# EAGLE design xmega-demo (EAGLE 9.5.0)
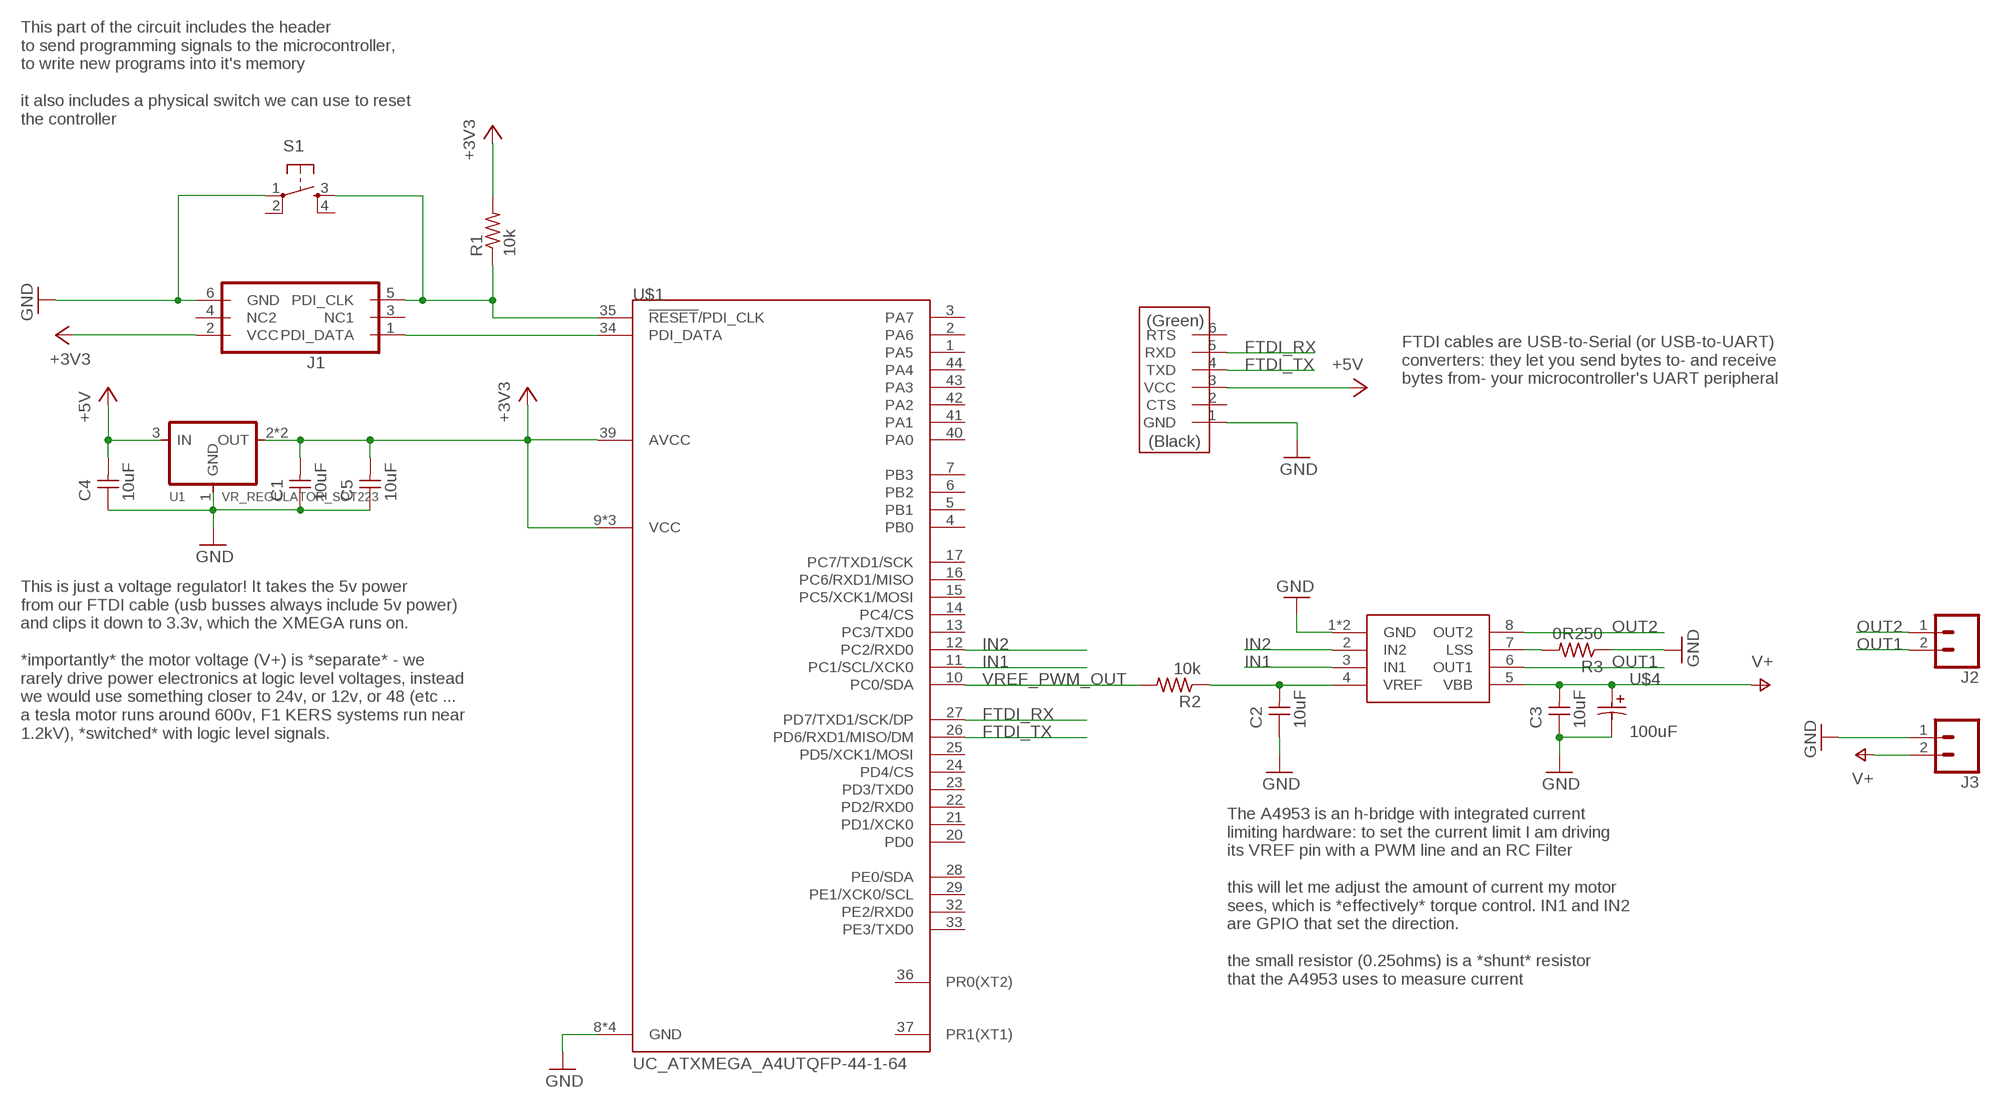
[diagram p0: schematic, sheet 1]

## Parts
C1  10uF  CAP_UNPOLARIZEDFAB  [C1206FAB]
C2  10uF  CAP_UNPOLARIZEDFAB  [C1206FAB]
C3  10uF  CAP_UNPOLARIZEDFAB  [C1206FAB]
C4  10uF  CAP_UNPOLARIZEDFAB  [C1206FAB]
C5  10uF  CAP_UNPOLARIZEDFAB  [C1206FAB]
J1  CONN_03X2_PDIFEMALE_SMD  [PDI_2X3_SMD]
J2  CONN_02  [1X02]
J3  CONN_02  [1X02]
R1  10k  R1206FAB  [R1206FAB]
R2  10k  R1206FAB  [R1206FAB]
R3  0R250  R1206FAB  [R1206FAB]
S1  SW_SWITCH_TACTILE_6MM6MM_SWITCH  [6MM_SWITCH]
U1  VR_REGULATOR_SOT223  [SOT223]
U$1  UC_ATXMEGA_A4UTQFP-44-1-64  [TQFP44-13THIN]
U$2  CONN_06_FTDI-SMD-HEADER  [1X06SMD]
U$3  PMIC_H-BRIDGE_A4953_PAD  [SOIC8_PAD]
U$4  100uF  CAP_POLARIZED  [SMD-ELEC-CAP]

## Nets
+3V3: C1.2 C5.2 J1.2(VCC) R1.2 U1.2(OUT) U1.4(OUT) U$1.9(VCC) U$1.19(VCC) U$1.31(VCC) U$1.39(AVCC)
+5V: C4.2 U1.3(IN) U$2.3(VCC)
FTDI_RX: U$1.27(PD7/TXD1/SCK/DP) U$2.5(RXD)
FTDI_TX: U$1.26(PD6/RXD1/MISO/DM) U$2.4(TXD)
GND: C1.1 C2.1 C3.1 C4.1 C5.1 J1.6(GND) J3.1 R3.1 S1.1(P) U1.1(GND) U$1.8(GND) U$1.18(GND) U$1.30(GND) U$1.38(GND) U$2.1(GND) U$3.1(GND) U$3.GND U$4.C
IN1: U$1.11(PC1/SCL/XCK0) U$3.3(IN1)
IN2: U$1.12(PC2/RXD0) U$3.2(IN2)
N$1: J1.1(PDI_DATA) U$1.34(PDI_DATA)
N$2: J1.5(PDI_CLK) R1.1 S1.3(S) U$1.35(!RESET!/PDI_CLK)
N$3: C2.2 R2.1 U$3.4(VREF)
N$5: R3.2 U$3.7(LSS)
OUT1: J2.2 U$3.6(OUT1)
OUT2: J2.1 U$3.8(OUT2)
V+: C3.2 J3.2 U$3.5(VBB) U$4.A
VREF_PWM_OUT: R2.2 U$1.10(PC0/SDA)
Unconnected: J1.3(NC1) J1.4(NC2) S1.2(P1) S1.4(S1) U$1.1(PA5) U$1.2(PA6) U$1.3(PA7) U$1.4(PB0) U$1.5(PB1) U$1.6(PB2) U$1.7(PB3) U$1.13(PC3/TXD0) U$1.14(PC4/CS) U$1.15(PC5/XCK1/MOSI) U$1.16(PC6/RXD1/MISO) U$1.17(PC7/TXD1/SCK) U$1.20(PD0) U$1.21(PD1/XCK0) U$1.22(PD2/RXD0) U$1.23(PD3/TXD0) U$1.24(PD4/CS) U$1.25(PD5/XCK1/MOSI) U$1.28(PE0/SDA) U$1.29(PE1/XCK0/SCL) U$1.32(PE2/RXD0) U$1.33(PE3/TXD0) U$1.36(PR0(XT2)) U$1.37(PR1(XT1)) U$1.40(PA0) U$1.41(PA1) U$1.42(PA2) U$1.43(PA3) U$1.44(PA4) U$2.2(CTS) U$2.6(RTS)

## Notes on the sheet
- This part of the circuit includes the header
  to send programming signals to the microcontroller,
  to write new programs into it's memory
  
  it also includes a physical switch we can use to reset 
  the controller
- FTDI cables are USB-to-Serial (or USB-to-UART) 
  converters: they let you send bytes to- and receive 
  bytes from- your microcontroller's UART peripheral
- This is just a voltage regulator! It takes the 5v power 
  from our FTDI cable (usb busses always include 5v power)
  and clips it down to 3.3v, which the XMEGA runs on.
  
  *importantly* the motor voltage (V+) is *separate* - we
  rarely drive power electronics at logic level voltages, instead
  we would use something closer to 24v, or 12v, or 48 (etc ...
  a tesla motor runs around 600v, F1 KERS systems run near 
  1.2kV), *switched* with logic level signals.
- The A4953 is an h-bridge with integrated current
  limiting hardware: to set the current limit I am driving 
  its VREF pin with a PWM line and an RC Filter
  
  this will let me adjust the amount of current my motor 
  sees, which is *effectively* torque control. IN1 and IN2 
  are GPIO that set the direction. 
  
  the small resistor (0.25ohms) is a *shunt* resistor
  that the A4953 uses to measure current

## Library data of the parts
C1-C5 = fablab:CAP_UNPOLARIZED
J1 = fablab:CONN_03X2_PDI: Multi connection point. Often used as Generic Header-pin footprint for 0.1 inch spaced/style header connections You can populate with any combo of single row headers, but if you'd like an exact match, check these: Header - 2x3 (Male, 0.1") (PRT-12807) Header - 2x3 (Female, 0.1") (PRT-13010) 2x3 Pin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; PROD_ID: CONN-11290
J2 J3 = SparkFun-Connectors:CONN_02: Multi connection point. Often used as Generic Header-pin footprint for 0.1 inch spaced/style header connections
R1-R3 = fablab:R: Resistor (US Symbol)
S1 = fablab:SW_SWITCH_TACTILE_6MM: OMRON SWITCH
U1 = fablab:VR_REGULATOR_SOT223
U$1 = fablab:UC_ATXMEGA_A4U
U$2 = fablab:CONN_06_FTDI-SMD-HEADER
U$3 = fablab:PMIC_H-BRIDGE_A4953_PAD
U$4 = fablab:CAP_POLARIZED

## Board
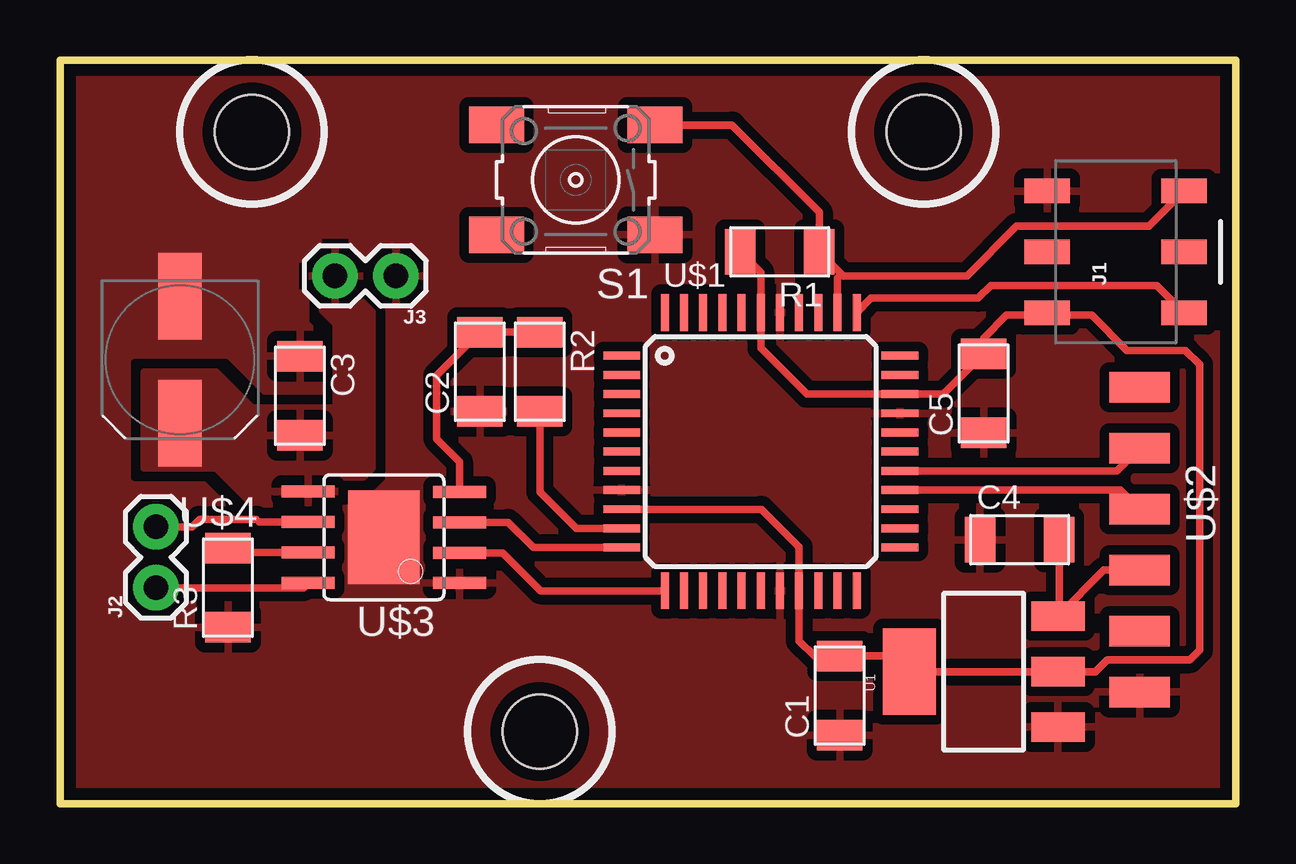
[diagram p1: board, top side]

Size 49 x 31 mm. Coordinates in mm from the lower left corner, seen from the top.
Outline: 0,0 49,0 49,31 0,31 0,0
Copper layers (1*16): Top 0.035mm / dielectric 1.5mm / Bottom 0.035mm
Design rules "default *": minimum track width 12mil, minimum drill 32mil, track to track 16mil, track to pad 16mil, pad to pad 16mil, via to via 16mil, smd to smd 0mil, copper to edge 20mil, drill to drill 16mil, minimum pad ring 10mil, minimum via ring 8mil, stop-mask expansion 4mil, vias tented up to drill 0mil, thermal gap 17mil
Holes 3.1 mm at 20,3 8,28 36,28

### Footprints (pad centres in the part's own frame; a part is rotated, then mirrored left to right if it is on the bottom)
C1206FAB = smd 1.27 x 1.905: 1 -1.651,0; 2 1.651,0
PDI_2X3_SMD = smd 1.02 x 1.9: 1 -2.54,-2.85; 2 -2.54,2.85; 3 0,-2.85; 4 0,2.85; 5 2.54,-2.85; 6 2.54,2.85
1X02 = drill 1.016 pad 1.88: 1 0,0; 2 2.54,0
R1206FAB = smd 1.27 x 1.905: 1 -1.651,0; 2 1.651,0
6MM_SWITCH = smd 2.286 x 1.524: 1 -3.302,2.286; 2 3.302,2.286; 3 -3.302,-2.286; 4 3.302,-2.286
SOT223 = smd 1.219 x 2.235: 1 -2.311,-3.099; 2 0,-3.099; 3 2.311,-3.099 | smd 3.6 x 2.2: 4 0,3.099
TQFP44-13THIN = smd 1.524 x 0.33: 1 -5.8,4; 2 -5.8,3.2; 3 -5.8,2.4; 4 -5.8,1.6; 5 -5.8,0.8; 6 -5.8,0; 7 -5.8,-0.8; 8 -5.8,-1.6; 9 -5.8,-2.4; 10 -5.8,-3.2; 11 -5.8,-4; 23 5.8,-4; 24 5.8,-3.2; 25 5.8,-2.4; 26 5.8,-1.6; 27 5.8,-0.8; 28 5.8,0; 29 5.8,0.8; 30 5.8,1.6; 31 5.8,2.4; 32 5.8,3.2; 33 5.8,4 | smd 0.33 x 1.524: 12 -4,-5.8; 13 -3.2,-5.8; 14 -2.4,-5.8; 15 -1.6,-5.8; 16 -0.8,-5.8; 17 0,-5.8; 18 0.8,-5.8; 19 1.6,-5.8; 20 2.4,-5.8; 21 3.2,-5.8; 22 4,-5.8; 34 4,5.8; 35 3.2,5.8; 36 2.4,5.8; 37 1.6,5.8; 38 0.8,5.8; 39 0,5.8; 40 -0.8,5.8; 41 -1.6,5.8; 42 -2.4,5.8; 43 -3.2,5.8; 44 -4,5.8
1X06SMD = smd 2.54 x 1.27: 1 0,6.35; 2 0,3.81; 3 0,1.27; 4 0,-1.27; 5 0,-3.81; 6 0,-6.35
SOIC8_PAD = smd 0.5 x 2.2: 1 -1.905,-3.154; 2 -0.645,-3.154; 3 0.625,-3.154; 4 1.895,-3.154; 5 1.905,3.154; 6 0.635,3.154; 7 -0.635,3.154; 8 -1.905,3.154 | smd 3.886 x 2.997: GND 0,0
SMD-ELEC-CAP = smd 1.8 x 3.6: A 0,2.65; C 0,-2.65

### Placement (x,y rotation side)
C1  32.5,4.5 90 top
C2  17.5,18 90 top
C3  10,17 270 top
C4  40,11 0 top
C5  38.5,17.1 90 top
J1  44,23 90 top
J2  4,9 90 top
J3  14,22 180 top
R1  30,23 180 top
R2  20,18 270 top
R3  7,9 90 top
S1  21.5,26 180 top
U1  38.5,5.5 90 top
U$1  29.21,14.67 0 top
U$2  45,11 180 top
U$3  13.5,11.1 90 top
U$4  5,18.5 180 top

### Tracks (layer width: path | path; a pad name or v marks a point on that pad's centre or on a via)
+3V3
  Top 0.305: J1.2 41.05,20.35 | 41.05,20.35 43.01,20.35 44.47,18.89 46.91,18.89 47.5,18.3 47.5,6.4 47.1,6 43.65,6 43.16,5.5 U1.2 U1.4 34.75,6.15 C1.2 31.45,6.15 30.81,6.79 U$1.19 30.81,10.69 29.23,12.27 U$1.9 | 41.05,20.35 39.45,20.35 38.5,19.41 C5.2 36.82,17.07 U$1.31 31.13,17.07 29.21,18.99 U$1.39 29.21,22.14 R1.2
+5V
  Top 0.305: U$2.3 43.52,9.73 U1.3 41.65,7.86 C4.2
FTDI_RX
  Top 0.305: U$1.27 44.06,13.87 U$2.5
FTDI_TX
  Top 0.305: U$1.26 44.2,13.07 U$2.4
GND
  pour Top (rank 6): -1,-2 50,-2 50,32 -1,32
IN1
  Top 0.305: U$3.3 18.68,11.73 19.73,10.67 U$1.11
IN2
  Top 0.305: U$3.2 18.45,10.45 20.03,8.87 U$1.12
N$1
  Top 0.305: J1.1 45.71,21.6 38.8,21.6 38.27,21.07 33.81,21.07 U$1.34
N$2
  Top 0.305: J1.5 45.38,24.07 39.87,24.07 37.8,22 32.65,22 32.58,22.08 | 32.58,22.08 R1.1 31.65,24.65 28.01,28.29 S1.3 | U$1.35 32.41,21.91 32.58,22.08
N$3
  Top 0.305: R2.1 C2.2 15.7,17.85 15.7,15.2 16.65,14.25 U$3.4
N$5
  Top 0.305: U$3.7 7.19,10.46 R3.2
OUT1
  Top 0.305: J2.2 5.51,11.54 5.82,11.84 8.18,11.84 8.29,11.73 U$3.6
OUT2
  Top 0.305: U$3.8 10.15,9 J2.1
V+
  pour Top: 3.5,18 6.5,18 8,16.5 11.5,16.5 11.5,20 10.5,21 10.5,23 12.5,23 12.5,21 13,20.5 13,14 11.5,12.5 8,12.5 6.5,14 3.5,14
VREF_PWM_OUT
  Top 0.305: U$1.10 21.53,11.47 20,13 R2.2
